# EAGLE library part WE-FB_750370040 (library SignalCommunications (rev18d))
WE-FB Flyback Transformer suitable for LT3573/ LT3574/ LT3575/ LT3748 Characteristics easy design in solution less external components needed small board space low cost no optocoupler needed! long term reliability voltage control no aging same external parts for different output voltages easy design of custom power supply due to standard circuit and change of transformers and two components for feedback loop Isolation voltage up to 2.5 kV Applications Isolated power design Sensor interfaces Isolated telecom converters Power over Ethernet Details see: http://katalog.we-online.de/en/pbs/WE-FB_Linear? Updated 2014-07-07 2014 (C) Wurth Elektronik
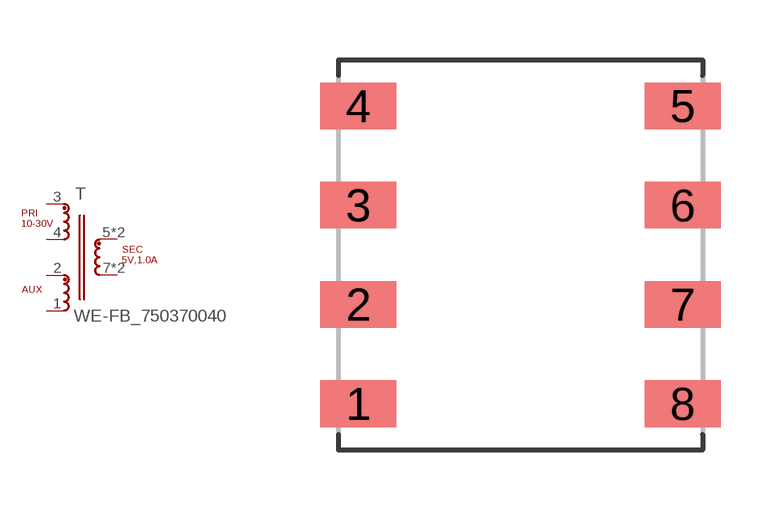
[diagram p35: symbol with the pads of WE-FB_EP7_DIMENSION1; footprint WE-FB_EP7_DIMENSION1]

Designator prefix T

## WE-FB_750370040  [WE-FB_EP7_DIMENSION1]
1  4  pas
2  5  pas
3  1  pas
4  6  pas
5  2  pas
6  2  pas
7  3  pas
8  3  pas

## Footprint WE-FB_EP7_DIMENSION1 (pad centres in mm)
Transformer, EP7* SMD 8Pin für WE-FB
smd 1.91 x 1.17: 1 -4.065,-3.735; 2 -4.065,-1.245; 3 -4.065,1.245; 4 -4.065,3.735; 5 4.065,3.735; 6 4.065,1.245; 7 4.065,-1.245; 8 4.065,-3.735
